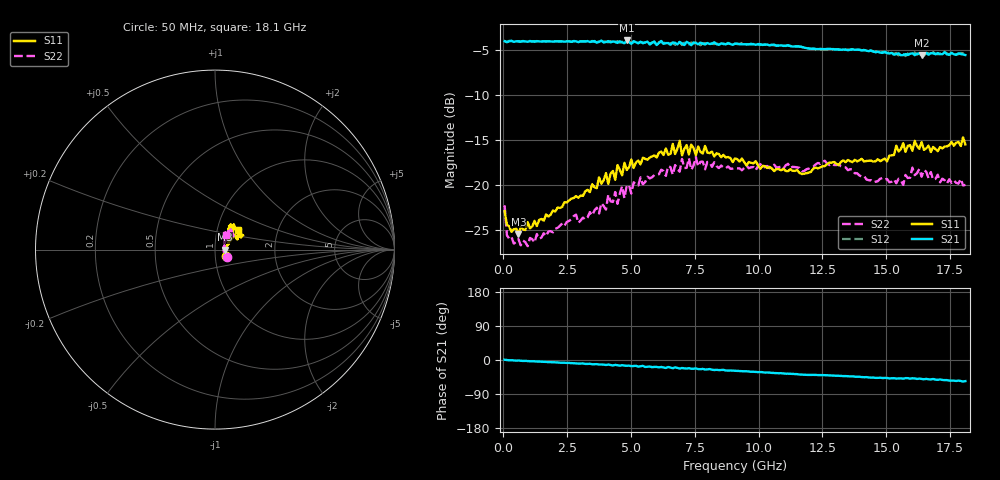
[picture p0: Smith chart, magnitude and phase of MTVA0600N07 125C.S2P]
! Network Analyzer HP8720D.06.14 Serial No. US36140669
!  6 Jul 2005  09:37:53
! Frequency  S11  S21  S12  S22
# HZ  S  DB R 50
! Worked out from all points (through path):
!   201 points, 50 MHz to 18.1 GHz, reference 50 ohm
!   highest |S21| = -3.91 dB at 4.833 GHz (marker M1); lowest = -5.6 dB at 16.39 GHz (marker M2)
!   group delay of S21, straight-line fit = 8.71 ps
!   lowest |S11| = -25.4 dB at 591.5 MHz (marker M3), VSWR 1.11, Z = 55.7 + j0.0595 ohm
!   |S11| at or under -10 dB: start of sweep to end of sweep
!   |S22| runs from -26.8 to -16.9 dB; largest |S21 - S12| = 0.027
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5e7  -22.88 -31.1  -3.99 0.7  -4.01 0.7  -22.23 -32.0
1.4025e8  -24.41 -17.1  -4.10 -0.0  -4.08 -0.2  -25.56 -18.2
5.915e8  -25.43 0.6  -3.99 -1.3  -4.06 -1.5  -25.99 2.8
9.525e8  -24.09 6.9  -4.05 -2.8  -3.98 -3.0  -26.78 7.8
3.1185e9  -21.18 29.9  -4.01 -9.1  -4.05 -9.4  -23.60 36.6
4.021e9  -18.66 37.8  -4.09 -13.1  -4.05 -12.2  -22.71 41.8
4.11125e9  -19.86 38.2  -3.98 -12.1  -4.11 -13.0  -21.04 43.2
4.47225e9  -17.76 36.8  -4.18 -13.8  -3.99 -13.5  -22.07 50.1
4.83325e9  -18.31 46.9  -3.91 -15.3  -4.11 -15.3  -20.04 42.6
6.09675e9  -16.38 47.9  -4.19 -19.4  -4.09 -19.3  -18.78 49.4
6.7285e9  -16.53 54.9  -4.17 -19.4  -4.39 -19.9  -17.76 46.9
6.909e9  -15.07 53.3  -4.07 -22.7  -4.11 -21.2  -18.49 47.3
6.99925e9  -16.69 53.1  -4.23 -21.0  -4.42 -22.5  -17.08 49.3
7.36025e9  -15.49 49.8  -4.44 -23.1  -4.16 -22.7  -18.29 53.2
7.54075e9  -16.68 51.7  -4.18 -22.1  -4.14 -24.5  -16.87 52.2
9.075e9  -17.02 55.7  -4.28 -28.4  -4.25 -28.6  -18.10 42.8
1.21435e10  -18.15 42.5  -4.84 -39.2  -4.79 -39.4  -17.93 51.3
1.512175e10  -16.72 28.9  -5.36 -48.6  -5.21 -48.2  -19.68 55.1
1.566325e10  -15.33 28.9  -5.53 -49.3  -5.43 -47.9  -19.97 53.5
1.602425e10  -16.17 27.8  -5.34 -48.3  -5.52 -50.1  -18.05 53.8
1.638525e10  -15.21 28.0  -5.56 -49.9  -5.34 -49.4  -19.06 52.0
1.81e10  -15.47 40.5  -5.54 -55.8  -5.67 -56.5  -19.96 52.9
